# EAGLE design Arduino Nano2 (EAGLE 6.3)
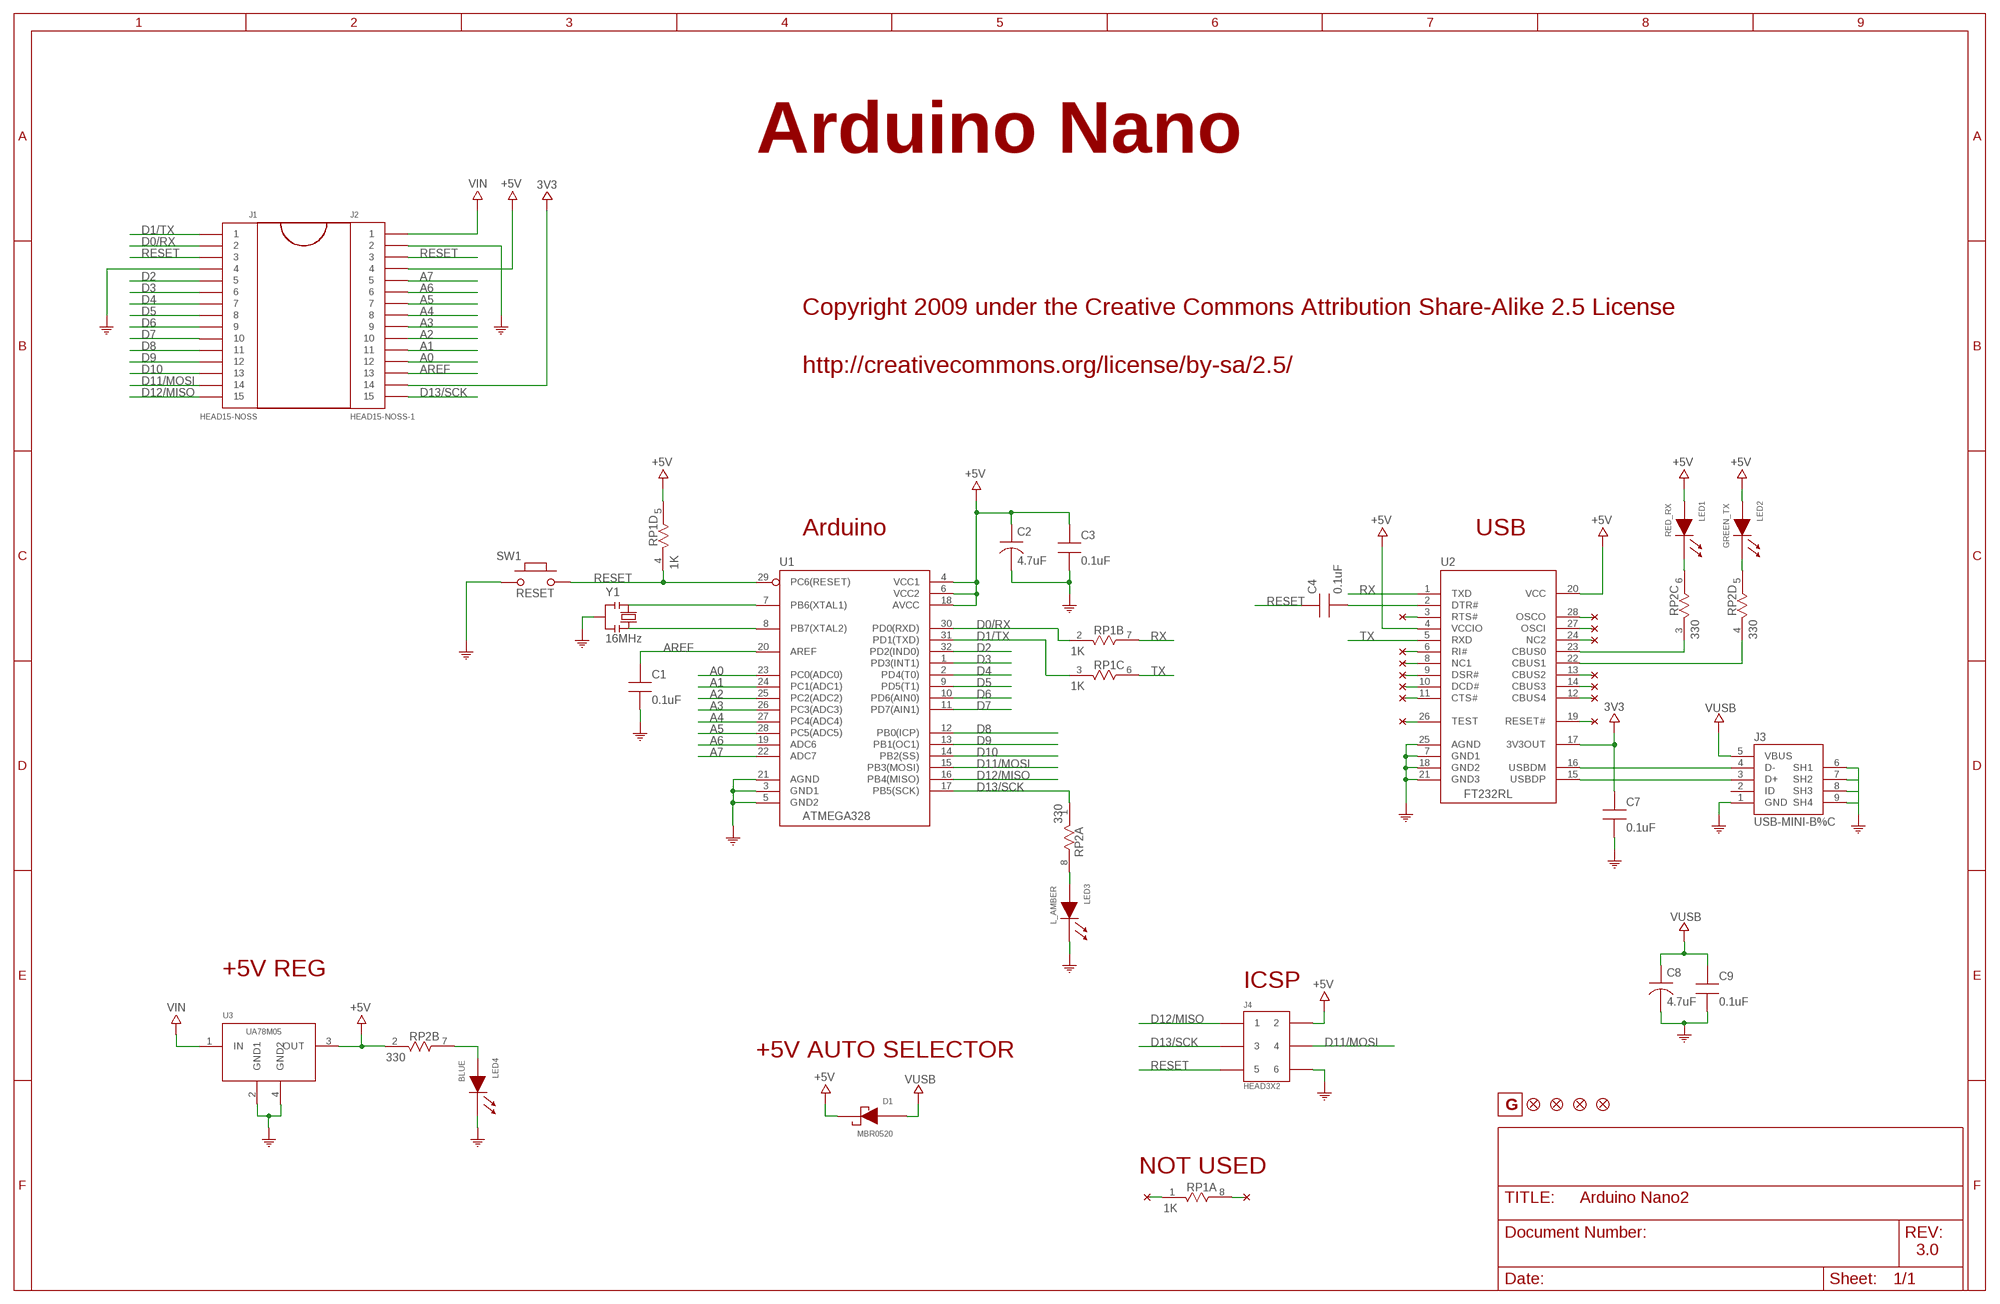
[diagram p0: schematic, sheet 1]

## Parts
C1  0.1uF  CAP0805-NP  [CAP0805-NP]
C2  4.7uF  CAP-TANA-P  [TAN-A]
C3  0.1uF  CAP0805-NP  [CAP0805-NP]
C4  0.1uF  CAP0805-NP  [CAP0805-NP]
C7  0.1uF  CAP0805-NP  [CAP0805-NP]
C8  4.7uF  CAP-TANA-P  [TAN-A]
C9  0.1uF  CAP0805-NP  [CAP0805-NP]
D1  MBR0520  [SOD-123]
J1  HEAD15-NOSS  [HEAD15-NOSS]
J2  HEAD15-NOSS-1  [HEAD15-NOSS-1]
J3  USB-MINI-B%C  [USB-MINI-B_2]
J4  HEAD3X2  [HEAD3X2]
LED1  RED_RX  LED0805  [LED0805]
LED2  GREEN_TX  LED0805  [LED0805]
LED3  L_AMBER  LED0805  [LED0805]
LED4  BLUE  LED0805  [LED0805]
RP1  1K  RES4NT  [RES4NT]
RP2  330  RES4NT  [RES4NT]
SW1  RESET  PB157  [157SW]
U1  ATMEGA328  ATMEGA168-20AU  [QFP032]
U2  FT232RL  [SSOP28]
U3  UA78M05  [SOT223]
U$4  FIDUCIAL1X2  [FIDUCIAL-1X2]
U$36  LOGO-G%117X105  [LOGO-G_117X105]
U$37  FIDUCIAL1X2  [FIDUCIAL-1X2]
U$53  FIDUCIAL1X2  [FIDUCIAL-1X2]
U$54  FIDUCIAL1X2  [FIDUCIAL-1X2]
Y1  16MHz  RESONATORMU  [RESONATOR]

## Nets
3V3: C7.1 J2.14 U2.17(3V3OUT)
+5V: C2.1 C3.1 D1.1(CA) J2.4 J4.2 LED1.2(AN) LED2.2(AN) RP1.5 RP2.2 U1.4(VCC1) U1.6(VCC2) U1.18(AVCC) U2.4(VCCIO) U2.20(VCC) U3.3(OUT)
A0: J2.12 U1.23(PC0(ADC0))
A1: J2.11 U1.24(PC1(ADC1))
A2: J2.10 U1.25(PC2(ADC2))
A3: J2.9 U1.26(PC3(ADC3))
A4: J2.8 U1.27(PC4(ADC4))
A5: J2.7 U1.28(PC5(ADC5))
A6: J2.6 U1.19(ADC6)
A7: J2.5 U1.22(ADC7)
AREF: C1.1 J2.13 U1.20(AREF)
COM: C1.2 C2.2 C3.2 C7.2 C8.2 C9.2 J1.4 J2.2 J3.1(GND) J3.6(SH1) J3.7(SH2) J3.8(SH3) J3.9(SH4) J4.6 LED3.1(CA) LED4.1(CA) SW1.1 U1.3(GND1) U1.5(GND2) U1.21(AGND) U2.7(GND1) U2.18(GND2) U2.21(GND3) U2.25(AGND) U3.2(GND1) U3.4(GND2) Y1.2
D0/RX: J1.2 RP1.2 U1.30(PD0(RXD))
D1/TX: J1.1 RP1.3 U1.31(PD1(TXD))
D2: J1.5 U1.32(PD2(IND0))
D3: J1.6 U1.1(PD3(INT1))
D4: J1.7 U1.2(PD4(T0))
D5: J1.8 U1.9(PD5(T1))
D6: J1.9 U1.10(PD6(AIN0))
D7: J1.10 U1.11(PD7(AIN1))
D8: J1.11 U1.12(PB0(ICP))
D9: J1.12 U1.13(PB1(OC1))
D10: J1.13 U1.14(PB2(SS))
D11/MOSI: J1.14 J4.4 U1.15(PB3(MOSI))
D12/MISO: J1.15 J4.1 U1.16(PB4(MISO))
D13/SCK: J2.15 J4.3 RP2.1 U1.17(PB5(SCK))
N$1: U1.8(PB7(XTAL2)) Y1.3
N$2: U1.7(PB6(XTAL1)) Y1.1
N$3: LED4.2(AN) RP2.7
N$4: C4.2 U2.2(DTR#)
N$5: J3.3(D+) U2.15(USBDP)
N$6: J3.4(D-) U2.16(USBDM)
N$7: LED3.2(AN) RP2.8
N$8: RP2.3 U2.23(CBUS0)
N$9: RP2.4 U2.22(CBUS1)
N$10: LED1.1(CA) RP2.6
N$11: LED2.1(CA) RP2.5
N$12: U2.11(CTS#)
N$13: U2.6(RI#)
N$14: U2.8(NC1)
N$15: U2.9(DSR#)
N$16: U2.10(DCD#)
N$17: U2.28(OSCO)
N$18: U2.27(OSCI)
N$19: U2.24(NC2)
N$20: U2.13(CBUS2)
N$21: U2.14(CBUS3)
N$22: U2.12(CBUS4)
N$23: U2.19(RESET#)
N$24: RP1.1
N$25: RP1.8
N$26: U2.26(TEST)
N$27: U2.3(RTS#)
RESET: C4.1 J1.3 J2.3 J4.5 RP1.4 SW1.2 U1.29(PC6(RESET))
RX: RP1.7 U2.1(TXD)
TX: RP1.6 U2.5(RXD)
VIN: J2.1 U3.1(IN)
VUSB: C8.1 C9.1 D1.2(AN) J3.5(VBUS)
Unconnected: J3.2(ID)

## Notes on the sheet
- Arduino Nano
- Copyright 2009 under the Creative Commons Attribution Share-Alike 2.5 License
- http://creativecommons.org/license/by-sa/2.5/
- Arduino | USB
- +5V REG
- ICSP
- +5V AUTO SELECTOR
- NOT USED
- 3.0

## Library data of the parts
C1 C3 C4 C7 C9 = MySMD:CAP0805-NP
C2 C8 = MySMD:CAP-TANA-P
D1 = MySMD:MBR0520
J1 = MyCON2:HEAD15-NOSS
J2 = MyCON2:HEAD15-NOSS-1
J3 = MyCON2:USB-MINI-B
J4 = MyCON2:HEAD3X2
LED1-LED4 = MySMD:LED0805
RP1 RP2 = MySMD:RES4NT
SW1 = MySMD:PB157
U1 = MySMD:ATMEGA168-20AU
U2 = MySMD2:FT232RL
U3 = MySMD:UA78M05
U$4 U$37 U$53 U$54 = SparkFun:FIDUCIAL: Fiducial Alignment Points
U$36 = MyBLK:LOGO-G
Y1 = MySMD2:RESONATOR

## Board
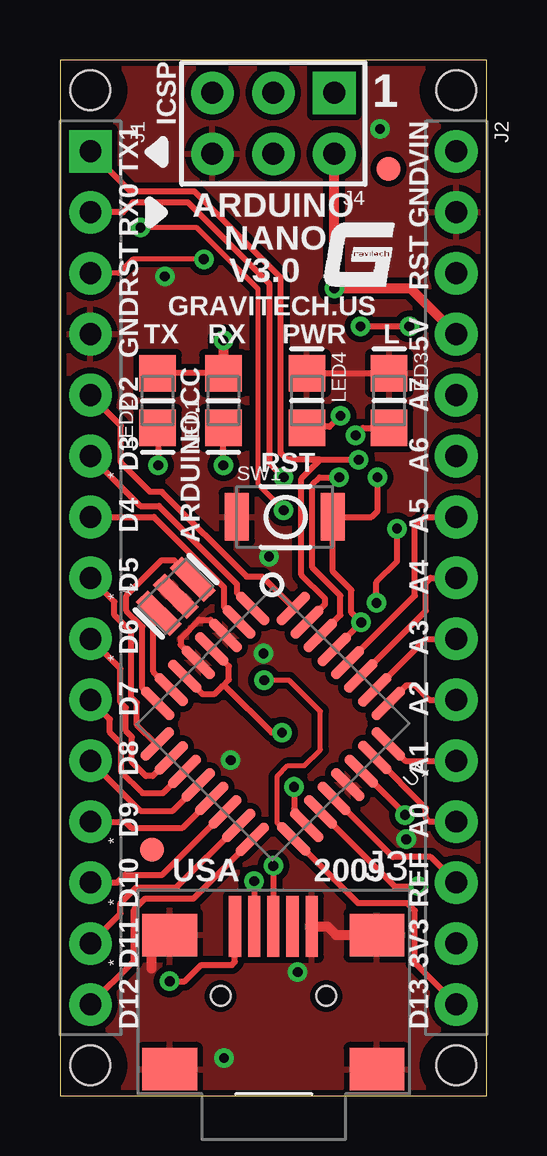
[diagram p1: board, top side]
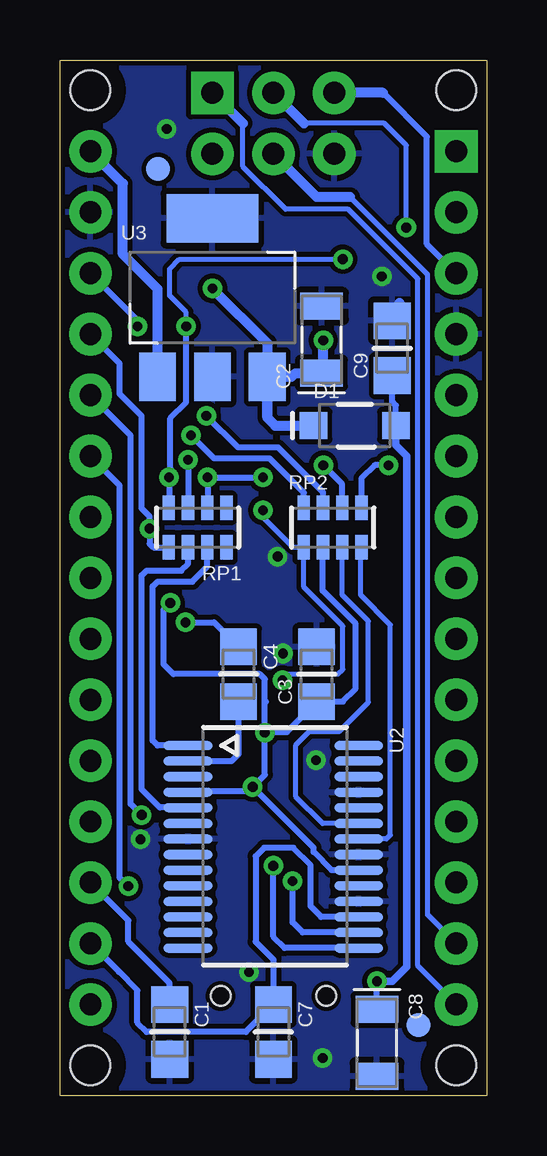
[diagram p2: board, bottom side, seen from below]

Size 17.78 x 43.18 mm. Coordinates in mm from the lower left corner, seen from the top.
Outline: 0,0 17.78,0 17.78,43.18 0,43.18 0,0
Copper layers (1*16): Top 0.035mm / dielectric 1.5mm / Bottom 0.035mm
Design rules "default *": minimum track width 8mil, minimum drill 16mil, track to track 8mil, track to pad 8mil, pad to pad 8mil, via to via 8mil, smd to smd 8mil, copper to edge 8mil, drill to drill 8mil, minimum pad ring 12mil, minimum via ring 8mil, stop-mask expansion 4mil, vias tented up to drill 18mil, thermal gap 10mil
Holes 1.65 mm at 1.27,1.27 16.51,1.27 16.51,41.91 1.27,41.91
tRestrict: area 0.1,0.1 to 2.4,2.4; area 15.4,40.8 to 17.7,43.1; area 15.4,0.1 to 17.7,2.4; area 0.1,40.8 to 2.4,43.1
bRestrict: area 15.4,0.1 to 17.7,2.4; area 0.1,0.1 to 2.4,2.4; area 0.1,40.8 to 2.4,43.1; area 15.4,40.8 to 17.7,43.1

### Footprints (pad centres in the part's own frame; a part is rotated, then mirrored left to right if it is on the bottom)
CAP0805-NP = smd 1.524 x 1.524: 1 0,0; 2 2.286,0
TAN-A = smd 1.118 x 1.778: 1 0,0; 2 2.794,0
SOD-123 = smd 1.143 x 1.143: 1 0,0; 2 3.429,0
HEAD15-NOSS = drill 0.914 pad 1.778 square: 1 0,0 | drill 0.914 pad 1.778: 2 2.54,0; 3 5.08,0; 4 7.62,0; 5 10.16,0; 6 12.7,0; 7 15.24,0; 8 17.78,0; 9 20.32,0; 10 22.86,0; 11 25.4,0; 12 27.94,0; 13 30.48,0; 14 33.02,0; 15 35.56,0
HEAD15-NOSS-1 = drill 0.914 pad 1.778: 1 0,0; 2 2.54,0; 3 5.08,0; 4 7.62,0; 5 10.16,0; 6 12.7,0; 7 15.24,0; 8 17.78,0; 9 20.32,0; 10 22.86,0; 11 25.4,0; 12 27.94,0; 13 30.48,0; 14 33.02,0; 15 35.56,0
USB-MINI-B_2 = smd 0.508 x 2.54: 1 0,0; 2 0.8,0; 3 1.6,0; 4 2.4,0; 5 3.2,0 | smd 2.286 x 1.778: 6 -2.717,5.948; 7 -2.717,0.36; 8 5.918,0.36; 9 5.918,5.948 | hole 0.813: -0.6,2.9; 3.8,2.9
HEAD3X2 = drill 0.914 pad 1.778 square: 1 0,0 | drill 0.914 pad 1.778: 2 0,2.54; 3 2.54,0; 4 2.54,2.54; 5 5.08,0; 6 5.08,2.54
LED0805 = smd 1.524 x 1.524: 1 0,0; 2 2.286,0
RES4NT = smd 0.508 x 1.016: 1 0,0; 2 0.8,0; 3 1.6,0; 4 2.4,0; 5 2.4,1.651; 6 1.6,1.651; 7 0.8,1.651; 8 0,1.651
157SW = smd 1.016 x 1.981: 1 0,0; 2 4,0
QFP032 = smd 0.432 x 1.778: 1 0,0; 2 0.8,0; 3 1.599,0; 4 2.399,0; 5 3.199,0; 6 3.998,0; 7 4.798,0; 8 5.598,0; 17 5.588,8.001; 18 4.798,7.997; 19 3.998,7.997; 20 3.199,7.997; 21 2.399,7.997; 22 1.599,7.997; 23 0.799,7.997; 24 0,7.997 | smd 1.778 x 0.432: 9 6.807,1.194; 10 6.807,2.007; 11 6.807,2.794; 12 6.807,3.607; 13 6.807,4.394; 14 6.807,5.182; 15 6.807,5.994; 16 6.816,6.803; 25 -1.194,6.807; 26 -1.194,5.994; 27 -1.194,5.182; 28 -1.194,4.394; 29 -1.194,3.607; 30 -1.194,2.794; 31 -1.194,2.007; 32 -1.194,1.194
SSOP28 = smd 0.381 x 2.032: 1 0,0; 2 0.65,0; 3 1.3,0; 4 1.95,0; 5 2.6,0; 6 3.25,0; 7 3.9,0; 8 4.55,0; 9 5.2,0; 10 5.85,0; 11 6.5,0; 12 7.15,0; 13 7.8,0; 14 8.45,0; 15 8.45,7.112; 16 7.8,7.112; 17 7.15,7.112; 18 6.5,7.112; 19 5.85,7.112; 20 5.2,7.112; 21 4.55,7.112; 22 3.9,7.112; 23 3.25,7.112; 24 2.6,7.112; 25 1.95,7.112; 26 1.3,7.112; 27 0.65,7.112; 28 0,7.112
SOT223 = smd 1.524 x 2.032: 1 0,0; 2 2.286,0; 3 4.572,0 | smd 3.81 x 2.032: 4 2.286,6.604
FIDUCIAL-1X2 = smd 1 x 1: 1 0,0
RESONATOR = smd 0.7 x 2: 1 -1,0; 2 0,0; 3 1,0

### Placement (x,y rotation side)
C1  13.21,3.81 270 bottom
C2  6.88,30.12 90 bottom
C3  7.09,16.43 90 bottom
C4  10.34,18.72 270 bottom
C7  8.89,3.81 270 bottom
C8  4.57,3.61 270 bottom
C9  3.94,30.02 90 bottom
D1  7.21,27.94 0 bottom
J1  1.27,39.37 270 top
J2  16.51,39.37 270 top
J3  10.49,7.06 180 top
J4  11.43,41.81 180 top
LED1  6.81,27.84 90 top
LED2  4.06,27.84 90 top
LED3  13.72,30.12 270 top
LED4  10.29,30.12 270 top
RP1  10.85,24.51 180 bottom
RP2  7.62,22.86 0 bottom
SW1  7.37,24.13 0 top
U1  8.03,20.32 225 top
U2  12.45,14.61 270 bottom
U3  13.72,29.97 0 bottom
U$4  13.69,38.63 0 top
U$36  12.57,35.05 0 top
U$37  3.84,10.26 0 top
U$53  13.69,38.63 0 bottom
U$54  2.84,2.95 0 bottom
Y1  4.83,20.83 45 top

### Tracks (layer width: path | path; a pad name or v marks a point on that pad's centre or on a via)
3V3
  Bottom 0.254: 15.34,5.18 J2.14 | 15.34,5.18 15.32,5.16 | U2.17 6.9,7.46 7.34,7.9 7.34,9.63 8.05,10.34 9.27,10.34 9.63,9.98 9.63,6.43 8.89,5.69 8.89,3.86 8.91,3.83 C7.1 10.03,2.67 14.17,2.67 14.55,3.05 14.55,4.39 15.34,5.18
+5V  (via drill 0.41, 0.41 pad 0.81)
  Top 0.254: LED1.2 LED2.2 | v9.75,12.88 9.75,11.96 U1.18 | v13.18,20.55 13.18,21.41 14.05,22.28 v14.05,23.65 | U1.6 5.94,16.74 6.43,16.74 6.76,17.07 | 6.76,17.07 7.04,17.35 7.04,17.91 U1.4 | 6.76,17.07 6.88,17.07 8.81,15.14 v9.25,15.14
  Top 0.406: v6.81,31.5 LED1.2 | J4.2 v11.43,33.66 14.61,33.66 J2.4
  Bottom 0.254: v9.75,12.88 9.93,12.7 11.46,12.7 U2.4 | v9.75,12.88 9.25,13.39 v9.25,15.14 | 9.25,16.46 9.25,17.37 9.45,17.58 13.06,17.58 13.46,17.98 13.46,20.27 v13.18,20.55 | 9.25,16.46 9.22,16.46 9.2,16.43 | J2.4 15.29,30.53 15.29,29.26 14.38,28.35 14.38,24.49 14.05,24.16 v14.05,23.65 14.05,23.01 13.89,22.86 RP1.5 | U2.20 6.46,9.4 7.21,10.16 7.21,10.34 v9.75,12.88 | v9.25,15.14 9.25,16.46 | v9.25,15.14 9.22,15.16 8.33,15.16 7.09,16.41 C3.1 5.99,16.43 5.46,16.97 5.46,19.68 6.83,21.06 6.83,22.84 6.82,22.85 RP2.2
  Bottom 0.406: 9.14,28.27 U3.3 8.13,29.97 7.98,30.12 C2.1 6.88,30.15 6.81,30.23 v6.81,31.5 | D1.1 8.81,27.94 9.14,28.27 | 9.14,28.27 9.14,31.37 v11.43,33.66
A0
  Top 0.254: U1.23 15.24,11.99 15.24,11.58 15.39,11.43 J2.12
A1
  Top 0.254: U1.24 14.38,13.97 J2.11
A2
  Top 0.254: U1.25 14.45,17.12 14.78,17.12 15.39,16.51 J2.10
A3
  Top 0.254: U1.26 15.24,19.05 J2.9
A4
  Top 0.254: U1.27 12.53,17.51 15.24,20.22 15.24,21.39 15.44,21.59 J2.8
A5
  Top 0.254: U1.28 14.78,20.85 14.78,23.72 15.19,24.13 J2.7
A6  (via drill 0.41 pad 0.81)
  Top 0.254: U1.19 10.89,11.84 10.89,11.79 13.95,8.74 v14.94,8.74
  Bottom 0.254: J2.6 15.29,25.45 15.29,9.09 v14.94,8.74
A7  (via drill 0.41 pad 0.81)
  Top 0.254: v14.38,11.71 14.38,11.73 12.58,13.53 U1.22
  Bottom 0.254: J2.5 14.83,27.53 14.83,12.17 v14.38,11.71
AREF
  Top 0.254: U1.20 13.87,9.96 15.44,9.96 J2.13
  Bottom 0.254: J2.13 14.94,7.32 14.94,6.43 13.21,4.7 C1.1
COM  (via drill 0.41, 0.41 pad 0.81)
  Top 0.254: LED4.1 LED3.1 | U1.5 5.03,18.8 5.03,19.07 5.79,19.84 6.27,19.84 6.89,19.22 U1.3
  Top 0.406: J3.1 11.15,7.06 11.51,6.71 J3.7 | J3.8 3.81,6.7 3.81,5.31
  Bottom 0.406: 3.63,33.05 3.83,32.84 C9.2
  other vias: 13.34,40.31 6.83,1.57 9.91,5.16 14.43,10.69 8.48,18.44 8.71,22.48 7.11,14 4.37,34.16
  pour Top (isolate 0.254): 0.25,0.25 0.25,42.93 17.53,42.93 17.53,0.25
  pour Bottom (isolate 0.203): 0.25,0.25 0.25,42.93 17.53,42.93 17.53,0.25
D0/RX  (via drill 0.41 pad 0.81)
  Top 0.254: U1.30 10.85,19.2 11.68,20.04 11.68,20.85 10.52,22.02 10.52,25.48 10.82,25.78 v11.63,25.78 | v9.32,25.78 8.74,26.36 8.74,33.83 5.33,37.24 3.02,37.24 2.62,36.83 J1.2
  Bottom 0.254: RP1.2 11.63,24.51 v11.63,25.78 v9.32,25.78
D1/TX  (via drill 0.41 pad 0.81)
  Top 0.254: U1.31 11.05,20.5 11.05,20.73 10.06,21.72 10.06,25.73 10.85,26.52 | 10.49,26.52 10.44,26.52 | 10.85,26.52 v12.45,26.52 | 10.85,26.52 10.49,26.52 | 10.49,26.52 9.47,26.52 9.2,26.8 9.2,34.11 5.61,37.69 2.95,37.69 J1.1
  Bottom 0.254: v12.45,26.52 RP1.3
D2
  Top 0.254: U1.32 9.71,20.36 8.43,21.64 7.77,21.64 4.24,25.17 3.76,25.17 2.54,26.39 2.54,27.94 J1.5
D3
  Top 0.254: U1.1 7.37,20.98 7.37,21.34 4.12,24.59 3.35,24.59 J1.6
D4
  Top 0.254: U1.2 7.46,19.77 6.83,20.4 6.83,21.21 3.91,24.13 J1.7
D5
  Top 0.254: U1.9 4.01,14.66 3.2,15.47 3.2,16.38 2.97,16.61 2.97,19.33 2.26,20.04 2.26,20.6 J1.8
D6
  Top 0.254: U1.10 4.61,14.09 3.86,13.34 3.58,13.34 3,13.92 3,14.96 2.74,15.21 2.74,16.18 2.52,16.41 2.52,17.8 J1.9
D7
  Top 0.254: U1.11 4.29,12.62 3.43,12.62 2.54,13.51 2.54,14.68 2.08,15.14 2.08,15.7 J1.10
D8
  Top 0.254: J1.11 3.35,11.89 4.7,11.89 U1.12
D9
  Top 0.254: U1.13 5.11,11.18 2.97,11.18 2.72,11.43 J1.12
D10
  Top 0.254: U1.14 4.27,9.22 2.72,9.22 2.39,8.89 J1.13
D11/MOSI
  Top 0.254: U1.15 4.85,8.69 3.17,8.69 2.52,8.03 2.52,7.59 J1.14
  Bottom 0.203: 5.69,37.47 2.46,34.24 2.46,7.54 J1.14
  Bottom 0.406: J4.4 7.09,37.47 5.69,37.47
D12/MISO
  Top 0.254: J1.15 3.07,5.61 3.07,7.75 3.56,8.23 5.56,8.23 U1.16 | U1.16 | U1.16
  Bottom 0.203: 10.16,40.54 10.16,38.73 8.38,36.96 5.77,36.96 2.87,34.06 2.87,5.41 J1.15
  Bottom 0.406: 10.16,40.54 J4.1
D13/SCK  (via drill 0.41 pad 0.81)
  Top 0.203: U1.17 9.71,10.71 9.04,11.38 9.04,13.31 9.5,13.77 10.19,13.77 10.85,14.43 10.85,16.03 9.55,17.32 v8.51,17.32 | v3.35,36.2 5.69,36.2 8.26,33.63 8.26,25.48 v9.32,24.41
  Top 0.254: U1.17 12.42,8.03 14.48,8.03 14.78,7.72 14.78,5.54 J2.15
  Bottom 0.203: v8.51,17.32 8.26,17.58 6.2,17.58 5.99,17.78 5.99,19.58 7.62,21.21 RP2.1 8.05,22.86 9.32,24.13 v9.32,24.41 | 7.62,40.54 4.27,40.54 3.35,39.62 v3.35,36.2
  Bottom 0.406: 7.62,40.54 J4.3
N$1
  Top 0.254: U1.8 4.07,16.38 4.04,16.38 3.43,16.99 3.43,19.56 2.77,20.22 2.77,20.85 4.24,22.33 4.75,22.33 Y1.3
N$2
  Top 0.254: U1.7 3.89,17.68 3.89,19.89 Y1.1
N$3  (via drill 0.41 pad 0.81)
  Top 0.254: LED4.2 10.34,27.84 10.39,27.89 11.23,27.89 v11.68,28.35
  Bottom 0.254: RP2.7 6.82,25.16 8.69,27.03 10.36,27.03 v11.68,28.35
N$4
  Bottom 0.254: U2.2 10.63,13.96 10.34,14.25 C4.2
N$5  (via drill 0.41 pad 0.81)
  Top 0.254: J3.3 8.89,9.45 v8.89,9.59
  Bottom 0.254: v8.89,9.59 8.89,6.63 8.42,6.16 5.35,6.16 U2.15
N$6  (via drill 0.41 pad 0.81)
  Top 0.254: J3.4 8.09,8.79 v8.09,8.95
  Bottom 0.254: v8.09,8.95 8.09,7.23 7.67,6.81 5.35,6.81 5.33,6.79 U2.16
N$7  (via drill 0.41 pad 0.81)
  Top 0.254: 13.74,27.84 LED3.2 12.62,27.84 v12.32,27.53
  Bottom 0.254: RP2.8 7.62,25.15 9.04,26.57 11.35,26.57 v12.32,27.53
N$8
  Bottom 0.203: U2.23 6.83,11.36 7.95,12.47 7.95,14.63 7.39,15.19 6.15,15.19 4.93,16.41 4.93,19.79 6.02,20.88 RP2.3
  Bottom 0.254: U2.23
N$9
  Bottom 0.203: U2.22 4.18,10.71 4.01,10.87 4.01,19.63 5.26,20.88 5.26,22.84 5.23,22.86 RP2.4
N$10  (via drill 0.41 pad 0.81)
  Top 0.254: 6.81,27.86 LED1.1 v6.81,26.29
  Bottom 0.254: RP2.6 6.02,25.5 v6.81,26.29
N$11  (via drill 0.41 pad 0.81)
  Top 0.254: LED2.1 v4.09,26.29
  Bottom 0.254: RP2.5 5.22,25.74 4.67,26.29 v4.09,26.29
RESET  (via drill 0.41, 0.41 pad 0.81)
  Top 0.203: v5.99,34.87 3.02,34.87 2.44,34.29 J1.3
  Top 0.254: U1.29 v12.55,19.74 12.14,20.14 12.14,21.08 11.37,21.86 SW1.2 12.98,24.13 13.23,24.38 v13.23,25.78 | v12.52,32.08 v14.55,32.08
  Bottom 0.203: v12.52,32.08 12.52,32.66 13.21,33.35 13.21,34.47 12.8,34.87 v5.99,34.87
  Bottom 0.254: 12.42,19.61 v12.55,19.74 11.35,19.74 C4.1 | RP1.4 13.23,24.54 v13.23,25.78 13.18,26.16 13.18,28.25 12.52,28.91 v12.52,32.08 | v14.55,32.08 14.55,32.33 J2.3 | J1.3 2.49,35.51 2.49,39.98 4.32,41.81
  Bottom 0.406: 4.32,41.81 J4.5
RX
  Bottom 0.254: RP1.7 11.65,22.06 12.27,21.44 13.72,21.44 13.92,21.23 13.92,14.81 13.72,14.61 U2.1
TX
  Bottom 0.254: RP1.6 12.45,22.17 12.72,21.89 14.17,21.89 14.38,21.69 14.38,12.78 13.61,12.01 12.45,12.01 U2.5
VIN
  Bottom 0.406: U3.1 13.72,33.63 15.16,35.08 15.16,38.02 J2.1
VUSB  (via drill 0.41 pad 0.81)
  Top 0.254: J3.5 7.29,5.59 7.16,5.46 5.89,5.46 5.21,4.78 v4.57,4.78
  Bottom 0.254: C8.1 v4.57,4.78 | D1.2 3.79,28.78 3.94,28.93 C9.1
  Bottom 0.305: v4.57,4.78 3.94,4.78 3.33,5.38 3.33,26.67 3.79,27.13 D1.2

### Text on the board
tPlace: 1 | ICSP | VIN | TX1 | ARDUINO | RX0 | GND | NANO | V3.0 | RST | RST | GRAVITECH.US | GND | TX | RX | PWR | L | 5V | D2 | A7 | * | D3 | RST | A6 | D4 | ARDUINO.CC | A5 | * | D5 | A4 | * | D6 | A3 | D7 | A2 | D8 | A1 | D9 | A0 | * | USA | 2009 | * | D10 | REF | * | D11 | 3V3 | D12 | D13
